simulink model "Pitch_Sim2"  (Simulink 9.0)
settings: Solver=ode45  StartTime=0.0  StopTime=100  RelTol=1e-3  EnableMultiTasking=on
InitFcn:
  | init
StartFcn:
  | init
StopFcn:
  | pl
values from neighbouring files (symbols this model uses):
  Cza = -0.032    [init.m]    (also in init_pitch.m)
  Czde = -0.0087    [init.m]    (also in init_pitch.m)
  d2r = 1/r2d    (= 0.0174532925199)    [freq.m]    (also in init.m; frequ.m; init_lat.m; pl.m)
  Mv = 1219.1    [init.m]    (also in init_lat.m; init_pitch.m)
  Qbar = 1220.6    [init.m]    (also in init_lat.m; init_pitch.m)
  r2d = 180/pi    (= 57.2957795131)    [freq.m]    (also in init.m; frequ.m; init_lat.m; pl.m)
  Sref = 145.4    [init.m]    (also in init_lat.m; init_pitch.m)
undefined symbols (not defined in the file or in its folder): Ap, Bp, Cp, Dp

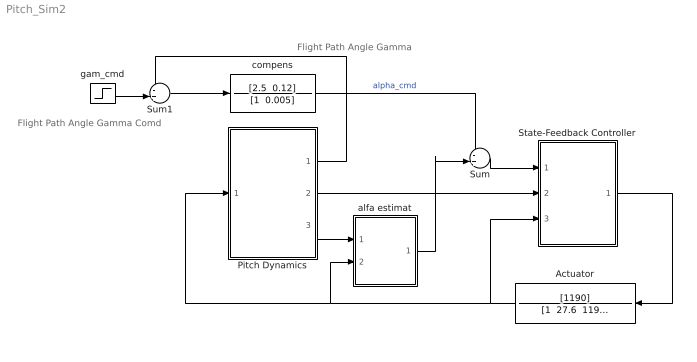
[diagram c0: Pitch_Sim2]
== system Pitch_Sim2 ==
  note: Flight Path Angle Gamma Comd
  note: Flight Path Angle Gamma
  Actuator : TransferFcn  Numerator=[1190]  Denominator="[1  27.6  1190]"
  Pitch Dynamics : Subsystem
  State-Feedback Controller : Subsystem
  Sum : Sum  Inputs=-+|
  Sum1 : Sum  Inputs=-+|
  alfa estimat : Subsystem
  compens : TransferFcn  Numerator="[2.5  0.12]"  Denominator="[1  0.005]"
  gam_cmd : Step  Time=0  After=d2r  SampleTime=0
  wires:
  Pitch Dynamics/2(q) -> State-Feedback Controller/2(q)
  Sum/1 -> State-Feedback Controller/1(alfa)
  compens/1 -> Sum/1  "alpha_cmd"
  Sum1/1 -> compens/1
  State-Feedback Controller/1(delv_cmd) -> Actuator/1
  Pitch Dynamics/3(Nz) -> alfa estimat/1(Nz)
  alfa estimat/1(alf_est) -> Sum/2
  Actuator/1 -> State-Feedback Controller/3(d-elev), Pitch Dynamics/1(elev), alfa estimat/2(d-elev)
  Pitch Dynamics/1(gamma) -> Sum1/1
  gam_cmd/1 -> Sum1/2

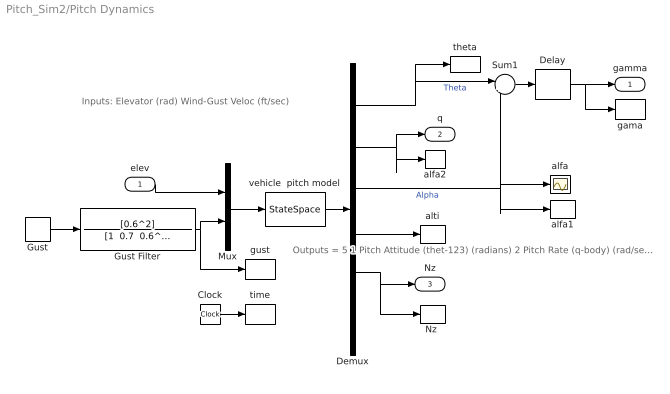
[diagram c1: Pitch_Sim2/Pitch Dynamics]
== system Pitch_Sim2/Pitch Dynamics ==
  note: Inputs: Elevator (rad) Wind-Gust Veloc (ft/sec)
  note: Outputs = 5 1 Pitch Attitude (thet-123) (radians) 2 Pitch Rate (q-body) (rad/sec) 3 Angle of attack, alfa, (radians) 4 Change in Altitude, delta-H, (feet) 5 Z-Acceleromet, (ft/sec^2) Translation 6 Alpha Sensed at Vane (radian)
  elev : Inport
  Clock : Clock
  Delay : TransportDelay  DelayTime=0.7  PadeOrder=2
  Demux : Demux  Outputs=6
  Gust : DiscretePulseGenerator  PulseType=Time based  Amplitude=30  Period=500  PulseWidth=2  PhaseDelay=10
  Gust Filter : TransferFcn  Numerator=[0.6^2]  Denominator="[1  0.7  0.6^2]"
  Mux : Mux  Inputs=2
  "Nz " : ToWorkspace  VariableName=Nz  SampleTime=-1
  Sum1 : Sum  Inputs=|+-
  alfa : Scope
  alfa1 : ToWorkspace  VariableName=alfa  SampleTime=-1
  alfa2 : ToWorkspace  VariableName=q  SampleTime=-1
  alti : ToWorkspace  VariableName=dH  SampleTime=-1
  gama : ToWorkspace  VariableName=gama  SampleTime=-1
  gust : ToWorkspace  VariableName=Vgst  SampleTime=-1
  theta : ToWorkspace  VariableName=theta  SampleTime=-1
  time : ToWorkspace  VariableName=time  SampleTime=-1
  vehicle  pitch model : StateSpace  A=Ap  B=Bp  C=Cp  D=Dp  InitialCondition=0
  gamma : Outport
  q : Outport  Port=2
  Nz : Outport  Port=3
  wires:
  Mux/1 -> vehicle  pitch model/1
  Demux/2 -> alfa2/1, q/1
  elev/1 -> Mux/1
  Demux/3 -> Sum1/2, alfa/1, alfa1/1  "Alpha"
  Demux/5 -> Nz/1, "Nz "/1
  Sum1/1 -> Delay/1
  Demux/1 -> Sum1/1, theta/1  "Theta"
  Gust Filter/1 -> Mux/2, gust/1
  Clock/1 -> time/1
  vehicle  pitch model/1 -> Demux/1
  Demux/4 -> alti/1
  Delay/1 -> gamma/1, gama/1
  Gust/1 -> Gust Filter/1

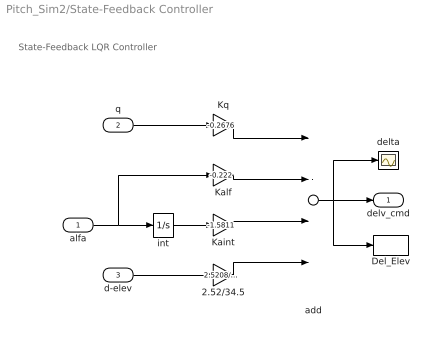
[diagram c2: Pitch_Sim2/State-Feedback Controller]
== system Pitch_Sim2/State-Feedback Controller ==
  note: State-Feedback LQR Controller
  alfa : Inport
  q : Inport  Port=2
  d-elev : Inport  Port=3
  2.52/34.5 : Gain  Gain=2.5208/34.5
  Del_Elev : ToWorkspace  VariableName=delev  SampleTime=-1
  Kaint : Gain  Gain=-1.5811
  Kalf : Gain  Gain=-0.222
  Kq : Gain  Gain=-0.2676
  add : Sum  Inputs=----
  delta : Scope
  int : Integrator
  delv_cmd : Outport
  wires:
  add/1 -> Del_Elev/1, delta/1, delv_cmd/1
  q/1 -> Kq/1
  d-elev/1 -> 2.52/34.5/1
  2.52/34.5/1 -> add/4
  Kaint/1 -> add/3
  Kalf/1 -> add/2
  Kq/1 -> add/1
  int/1 -> Kaint/1
  alfa/1 -> Kalf/1, int/1

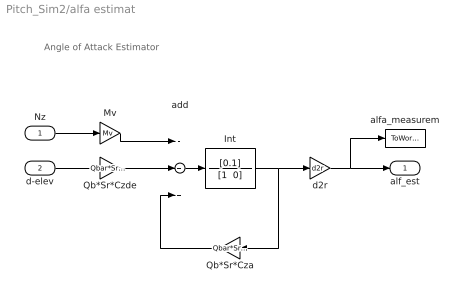
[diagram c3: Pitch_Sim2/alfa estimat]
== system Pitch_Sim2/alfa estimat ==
  note: Angle of Attack Estimator
  Nz : Inport
  d-elev : Inport  Port=2
  Int : TransferFcn  Numerator=[0.1]  Denominator="[1  0]"
  Mv : Gain  Gain=Mv
  Qb*Sr*Cza : Gain  Gain=Qbar*Sref*Cza
  Qb*Sr*Czde : Gain  Gain=Qbar*Sref*Czde*r2d
  add : Sum  Inputs=-++
  alfa_measurem : ToWorkspace  VariableName=alfa_est  SampleTime=-1
  d2r : Gain  Gain=d2r
  alf_est : Outport
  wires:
  add/1 -> Int/1
  Qb*Sr*Cza/1 -> add/3
  Mv/1 -> add/1
  Qb*Sr*Czde/1 -> add/2
  d2r/1 -> alf_est/1, alfa_measurem/1
  Int/1 -> Qb*Sr*Cza/1, d2r/1
  d-elev/1 -> Qb*Sr*Czde/1
  Nz/1 -> Mv/1
